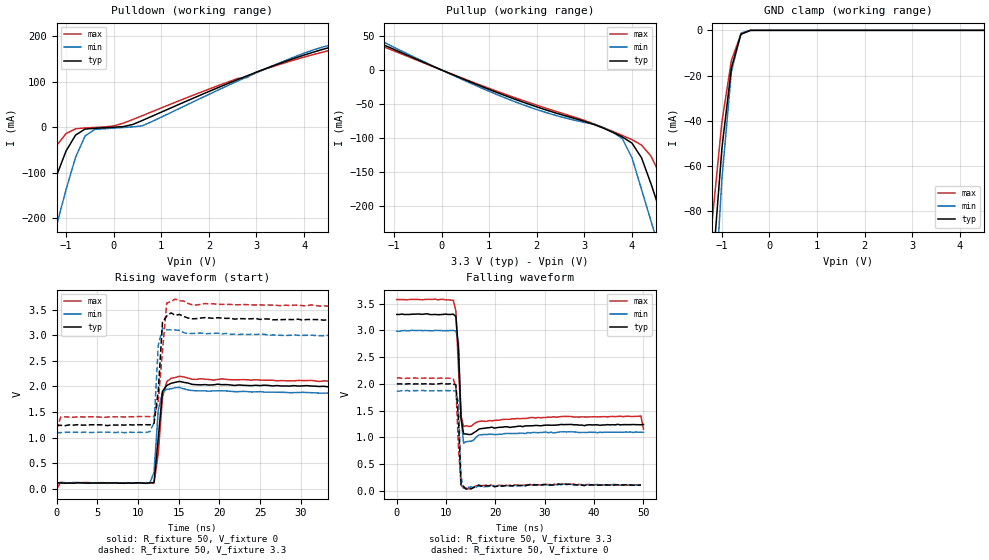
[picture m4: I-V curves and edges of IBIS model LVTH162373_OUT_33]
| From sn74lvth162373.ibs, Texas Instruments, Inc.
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|  Model LVTH162373 OUTPUT_33
[Model]   LVTH162373_OUT_33
Model_type  3-state
Polarity   Non-Inverting
Enable   Active-Low
Vmeas = 1.5V
Cref = 50pF
Rref = 500
Vref = 0
| variable   typ   min   max
C_comp   9p   NA   NA
[Temperature Range]   25   -40   85
[Voltage range]   3.3   3.0   3.6
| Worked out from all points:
|   slope of the pulldown table from 0 to 0.495 V, typ, clamps not added: 49 ohm
|   slope of the pullup table from 0 to 0.495 V, typ, clamps not added: 34.2 ohm
|   GND clamp passes 1 mA (typ) near -0.52 V on its own axis
|   rising waveform, R_fixture 50, V_fixture 0: 20-80 % time 659ps typ, 455ps min, 705ps max; typ from 0.114 V to 2 V
|   falling waveform, R_fixture 50, V_fixture 3.3: 20-80 % time 608ps typ, 424ps min, 774ps max; typ from 3.3 V to 1.24 V
|   rising waveform, R_fixture 50, V_fixture 3.3: 20-80 % time 593ps typ, 391ps min, 858ps max; typ from 1.24 V to 3.3 V
|   falling waveform, R_fixture 50, V_fixture 0: 20-80 % time 595ps typ, 395ps min, 643ps max; typ from 2 V to 0.111 V
[Pullup]
|   25C:3.3V   -40C:3.0V   85C:3.6V
|   Voltage   I(typ)   I(min)   I(max)
-5V       93.84uA    87.31uA    104.4uA
-2V       82.58uA    72.12uA    89.52uA
-1.8V     82.11uA    60.8mA     89.03uA
-1.6V     81.63uA    54.13mA    88.54uA
-1.4V     81.13uA    46.72mA    39.47mA
-1.2V     36.55mA    40.75mA    33.85mA
3.6V      -92.04mA   -91.8mA    -90.74mA
4.2V      -129.5mA   -176.4mA   -110.7mA
4.4V      -168.1mA   -223.2mA   -127.2mA
4.6V      -210.8mA   -270mA     -156.1mA
5V        -296.2mA   -363.6mA   -240.4mA
10V       -1.364A    -1.534A    -1.294A
[Pulldown]
|   25C:3.3V   -40C:3.0V   85C:3.6V
|   Voltage   I(typ)   I(min)   I(max)
-5V       -1.588A    -1.723A    -1.352A
-1.8V     -341mA     -454.5mA   -220mA
-1.6V     -263mA     -375.3mA   -149.2mA
-1.4V     -185.1mA   -296mA     -82.69mA
-1.2V     -107.1mA   -216.7mA   -40.6mA
-800mV    -17.47mA   -66.35mA   -3.608mA
-600mV    -4.261mA   -19.46mA   -1.81mA
-400mV    -2.553mA   -4.942mA   -704uA
600mV     14.57mA    2.87mA     25.22mA
4.4V      171.5mA    176.6mA    165.3mA
6.6V      212.9mA    220mA      200.4mA
10V       265.2mA    281.9mA    233mA
[GND Clamp]
|   25C:2.8V   -40C:2.7V   85C:2.9V
|   Voltage   I(typ)   I(min)   I(max)
-5V       -1.686A    -1.93A     -1.49A
-1.4V     -187.1mA   -231mA     -150.5mA
-1.2V     -106.9mA   -136.6mA   -83.49mA
-1V       -52.29mA   -65.87mA   -40.6mA
-800mV    -16.54mA   -18.25mA   -13.27mA
-600mV    -1.712mA   -1.24mA    -1.686mA
-400mV    -7.76uA    -3.295uA   -12.98uA
5V        24.55nA    164nA      156.6nA
[ramp]
| variable   typ   min   max
dV/dt_r   1.146E+00/3.650E-10  1.068E+00/3.800E-10  1.218E+00/4.370E-10
dV/dt_f   1.242E+00/5.520E-10  1.152E+00/4.440E-10  1.338E+00/5.710E-10
R_load = 50
[Rising Waveform]
R_fixture = 50
V_fixture = 0
V_fixture_min = 0
V_fixture_max = 0
C_fixture = 0
L_fixture = 0
|   25C:3.3V   -40C:3.0V   85C:3.6V
|   Time   V(typ)   V(min)   V(max)
|   0.000E+00   1.144E-01   1.123E-01   1.266E-01
0s        114.4mV    112.3mV    -8.4mV
520.8ps   114.4mV    112.3mV    126.6mV
11.46ns   113.5mV    110.3mV    118.3mV
11.98ns   121.8mV    324.1mV    111.2mV
12.5ns    991.1mV    1.538V     691.8mV
13.02ns   1.904V     1.882V     1.792V
13.54ns   2.017V     1.944V     2.091V
14.06ns   2.059V     1.952V     2.157V
46.88ns   2.003V     1.875V     2.115V
50ns      2.002V     1.882V     2.048V
[Falling Waveform]
R_fixture = 50
V_fixture = 3.3
V_fixture_min = 3.0
V_fixture_max = 3.6
C_fixture = 0
L_fixture = 0
|   25C:3.3V   -40C:3.0V   85C:3.6V
|   Time   V(typ)   V(min)   V(max)
0s        3.296V     2.983V     3.575V
11.46ns   3.302V     2.997V     3.561V
11.98ns   3.256V     2.988V     3.359V
12.5ns    2.634V     2.775V     2.293V
13.02ns   1.352V     1.389V     1.408V
13.54ns   1.068V     891.3mV    1.201V
15.1ns    1.057V     930mV      1.211V
17.71ns   1.171V     1.055V     1.302V
49.48ns   1.236V     1.098V     1.401V
50ns      1.243V     1.098V     1.153V
[Rising Waveform]
R_fixture = 50
V_fixture = 3.3
V_fixture_min = 3.0
V_fixture_max = 3.6
C_fixture = 0
L_fixture = 0
|   25C:3.3V   -40C:3.0V   85C:3.6V
|   Time   V(typ)   V(min)   V(max)
0s        1.239V     1.096V     1.158V
520.8ps   1.239V     1.096V     1.4V
10.94ns   1.252V     1.099V     1.412V
11.98ns   1.278V     1.286V     1.413V
12.5ns    1.915V     2.803V     1.708V
13.02ns   3.254V     3.137V     2.701V
13.54ns   3.376V     3.104V     3.626V
14.58ns   3.389V     3.102V     3.706V
17.19ns   3.324V     3.038V     3.589V
50ns      3.299V     2.998V     3.585V
[Falling Waveform]
R_fixture = 50
V_fixture = 0
V_fixture_min = 0
V_fixture_max = 0
C_fixture = 0
L_fixture = 0
|   25C:3.3V   -40C:3.0V   85C:3.6V
|   Time   V(typ)   V(min)   V(max)
0s        2V         1.865V     2.112V
11.46ns   1.995V     1.87V      2.093V
11.98ns   1.982V     1.868V     1.935V
12.5ns    1.331V     1.655V     821.5mV
13.02ns   122.2mV    271.2mV    114.1mV
13.54ns   84.99mV    52.49mV    52.34mV
14.06ns   34.18mV    42.11mV    53.25mV
16.67ns   110.5mV    94.45mV    104.1mV
18.75ns   95.52mV    85.6mV     113.8mV
49.48ns   110.8mV    114.4mV    112mV
